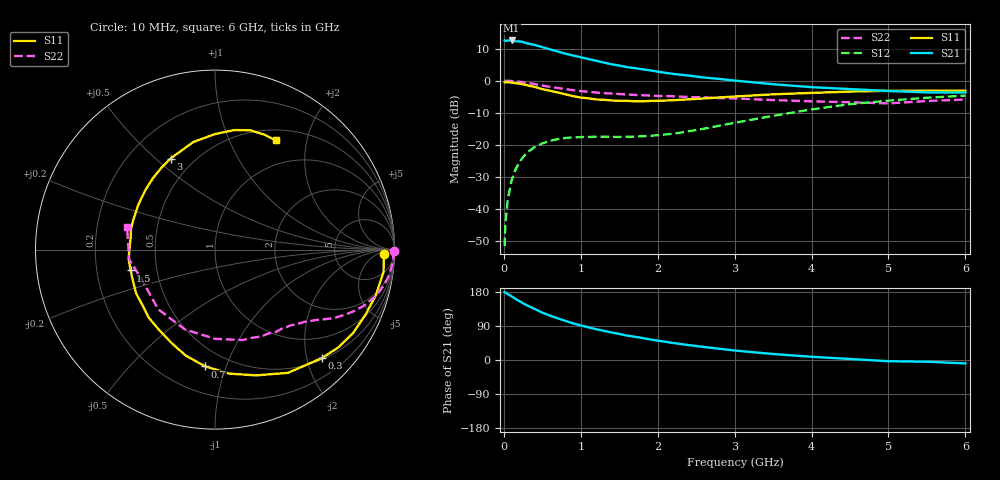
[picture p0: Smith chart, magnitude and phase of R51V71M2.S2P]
! SIEMENS Small Signal Semiconductors
! BFR183
! Si NPN RF Bipolar Junction Transistor in SOT23
! VCE = 1.75 V  IC = 1.2 mA
! Common Emitter S-Parameters:  May  1996
# GHz  S  MA  R  50
!  f  S11  S21  S12  S22
! GHz  MAG  ANG  MAG  ANG  MAG  ANG  MAG  ANG
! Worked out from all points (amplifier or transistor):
!   36 points, 10 MHz to 6 GHz, reference 50 ohm
!   highest |S21| = 12.6 dB at 100 MHz (marker M1)
!   |S21| within 3 dB of that: start of sweep to 633.1 MHz
!   unconditionally stable (mu >= 1): 1.576 GHz to 2.948 GHz
!   at 250 MHz: K = 0.17, MSG = 18.0 dB, |S12| = -23.9 dB
!   at 1.4 GHz: K = 0.91, MSG = 11.3 dB, |S12| = -17.6 dB
!   at 6 GHz: K = 0.95, MSG = 0.5 dB, |S12| = -4.7 dB
!   S11 on the Smith chart (normalised r, x): 10 MHz: 28, -13; 300 MHz: 0.53, -2.28; 700 MHz: 0.37, -0.85; 1.5 GHz: 0.35, -0.11; 3 GHz: 0.38, +0.56; 6 GHz: 0.64, +1.51
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0.01  0.9433 -1.6  4.229 179.2  0.0026 85.7  0.9985 -0.6
0.02  0.942 -3.2  4.161 177.5  0.0057 90.0  0.9903 -1.2
0.05  0.9471 -7.7  4.232 174.0  0.0136 85.4  0.9962 -3.1
0.1  0.9315 -15.8  4.242 168.1  0.0274 80.9  0.9867 -6.1
0.15  0.9139 -23.3  4.105 161.4  0.0407 75.9  0.9774 -9.0
0.2  0.8992 -31.1  4.103 155.5  0.0528 71.7  0.9629 -11.7
0.25  0.8763 -38.6  4.002 149.8  0.064 67.5  0.9435 -14.5
0.3  0.8479 -45.5  3.827 144.3  0.0747 63.9  0.9249 -16.8
0.4  0.7979 -59.4  3.617 134.8  0.0919 56.9  0.8837 -20.9
0.5  0.7368 -72.0  3.336 124.9  0.1046 50.8  0.8389 -24.5
0.7  0.653 -94.8  2.857 109.9  0.1222 41.9  0.769 -29.6
0.9  0.573 -115.3  2.47 96.7  0.1301 36.4  0.7102 -33.2
1.1  0.5293 -134.3  2.177 86.2  0.1324 33.3  0.6687 -36.4
1.2  0.5086 -142.9  2.044 81.2  0.1326 32.4  0.6521 -37.9
1.5  0.4844 -166.1  1.721 68.9  0.1324 33.0  0.6177 -41.9
1.9  0.482 166.2  1.447 54.3  0.1371 39.7  0.5852 -48.1
2.2  0.4943 150.1  1.275 45.0  0.1479 45.2  0.5709 -53.4
3  0.5647 116.0  1.003 25.0  0.2194 54.0  0.527 -73.0
3.5  0.6115 101.4  0.879 15.8  0.282 52.0  0.4972 -89.9
4.5  0.6744 80.9  0.738 2.7  0.43 39.0  0.4588 -133.7
5.5  0.6973 66.4  0.655 -4.6  0.5412 22.8  0.4813 -173.4
6  0.6957 60.9  0.652 -9.0  0.5839 13.0  0.5066 165.4
